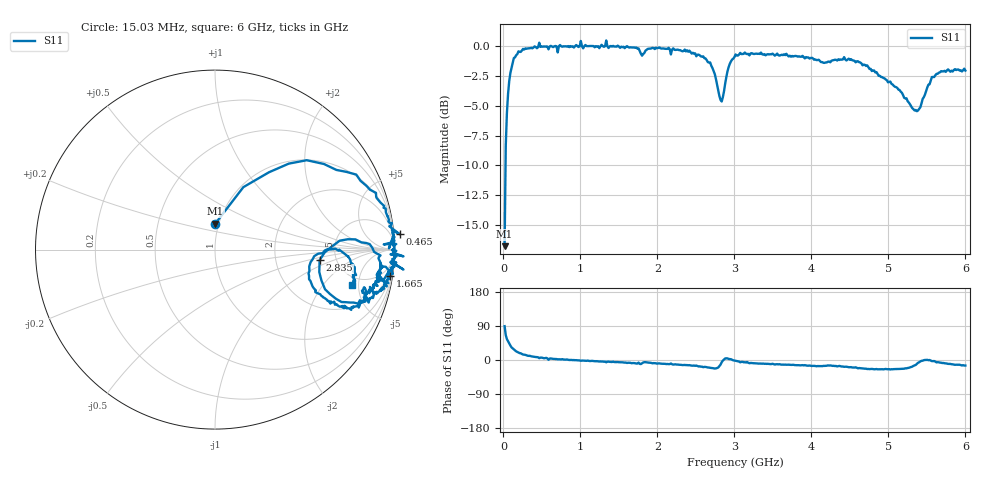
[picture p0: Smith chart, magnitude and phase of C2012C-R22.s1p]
!	Network	Analyzer	HP8753E.07.74:	Oct	30	2002	Serial	No.	JP38451487
!	Hewlett-Packard
!	7	Sep	2009	12:18:27
!	Frequency	S11
#	HZ	S	RI	R	50
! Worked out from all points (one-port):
!   400 points, 15.03 MHz to 6 GHz, reference 50 ohm
!   lowest |S11| = -16.8 dB at 15.03 MHz (marker M1), VSWR 1.34, Z = 48.1 + j14.3 ohm
!   |S11| at or under -10 dB: start of sweep to 27.1 MHz
!   S11 on the Smith chart (normalised r, x): 15.03 MHz: 0.96, +0.29; 465 MHz: -8, +21; 1.665 GHz: 1, -13; 2.835 GHz: 3.70, -0.66; 6 GHz: 3.95, -4.18
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1.502992e7  0.00192 0.145
3.002985e7  0.158 0.348
6.00297e7  0.411 0.479
9.002955e7  0.607 0.477
1.95029e8  0.897 0.316
4.650277e8  1.03 0.0851
7.650262e8  0.993 0.0387
1.005025e9  1.05 -0.0376
1.245024e9  0.978 -0.0687
1.335023e9  1.05 -0.111
1.515022e9  0.978 -0.101
1.665022e9  0.976 -0.145
1.800021e9  0.901 -0.14
2.265019e9  0.945 -0.201
2.625017e9  0.843 -0.278
2.745016e9  0.705 -0.292
2.835016e9  0.583 -0.0584
2.895016e9  0.74 0.0576
3.015015e9  0.922 -0.0324
3.195014e9  0.904 -0.136
3.765011e9  0.883 -0.197
4.515007e9  0.834 -0.285
4.815006e9  0.719 -0.327
5.265004e9  0.543 -0.204
5.370003e9  0.525 -0.0937
5.505002e9  0.671 0.00519
5.685002e9  0.779 -0.098
6e9  0.764 -0.199
